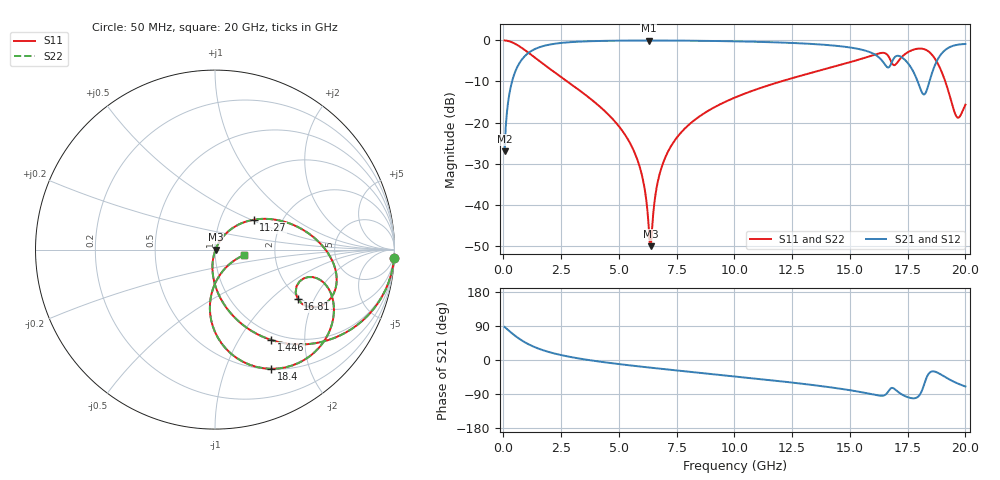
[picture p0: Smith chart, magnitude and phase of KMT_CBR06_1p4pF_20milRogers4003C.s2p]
! Data measured by Modelithics Inc. support@modelithics.com 813-866-6335
! KEMET CBR0603 1.4pF, Pad Width= 0.851mm, Pad Length= 0.64mm, Pad Gap= 0.62mm, 20mil Rogers 4003C substrate Data, January 2022
# hz S ma R 50
! 2 Port Network Data from SP1.SP block
! freq  magS11  angS11  magS21  angS21  magS12  angS12  magS22  angS22
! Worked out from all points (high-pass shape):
!   401 points, 50 MHz to 20 GHz, reference 50 ohm
!   highest |S21| = -0.03 dB at 6.284 GHz (marker M1); lowest = -27.0 dB at 50 MHz (marker M2)
!   |S21| within 3 dB of the highest: 1.087 GHz to 15.94 GHz (14.85 GHz wide, 174 % of centre); 19 GHz to end of sweep
!   lowest |S11| = -50.1 dB at 6.384 GHz (marker M3), VSWR 1.01, Z = 50.3 + j0.00703 ohm
!   |S11| at or under -10 dB: 2.763 GHz to 12.01 GHz (9.249 GHz wide, 125 % of centre); 19.13 GHz to end of sweep
!   |S22| runs from -50.1 to 0.0 dB; largest |S21 - S12| = 0
!   S11 on the Smith chart (normalised r, x): 50 MHz: 1, -42; 1.446 GHz: 0.89, -1.39; 11.27 GHz: 1.44, +0.52; 16.81 GHz: 1.94, -1.50; 18.4 GHz: 0.50, -1.45; 20 GHz: 1.38, -0.09
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5e7  0.999 -2.7  0.04465 87.3  0.04465 87.3  0.999 -2.7
4.98875e8  0.9121 -25.7  0.409 64.2  0.409 64.2  0.9121 -25.7
1.4465e9  0.5924 -58.1  0.804 31.7  0.804 31.7  0.5924 -58.1
3.391625e9  0.2348 -86.7  0.9697 2.8  0.9697 2.8  0.2348 -86.7
5.53625e9  0.0524 -101.6  0.9957 -14.6  0.9957 -14.6  0.0524 -101.6
6.035e9  0.02038 -100.1  0.9968 -18.0  0.9968 -18.0  0.02038 -100.1
6.284375e9  0.005651 -79.1  0.9969 -19.7  0.9969 -19.7  0.005651 -79.1
6.384125e9  0.003122 1.3  0.9969 -20.4  0.9969 -20.4  0.003122 1.3
6.73325e9  0.02195 59.6  0.9965 -22.6  0.9965 -22.6  0.02195 59.6
7.780625e9  0.08059 58.4  0.9933 -29.3  0.9933 -29.3  0.08059 58.4
1.0025e10  0.2018 45.6  0.9751 -43.3  0.9751 -43.3  0.2018 45.6
1.127188e10  0.272 37.7  0.9571 -51.3  0.9571 -51.3  0.272 37.7
1.336662e10  0.406 23.0  0.9054 -65.8  0.9054 -65.8  0.406 23.0
1.62095e10  0.689 -11.3  0.6372 -93.5  0.6372 -93.5  0.689 -11.3
1.670825e10  0.6136 -31.5  0.4758 -78.8  0.4758 -78.8  0.6136 -31.5
1.6808e10  0.5361 -30.8  0.5373 -73.6  0.5373 -73.6  0.5361 -30.8
1.770575e10  0.7637 -30.5  0.4381 -101.0  0.4381 -101.0  0.7637 -30.5
1.815462e10  0.7907 -51.0  0.2239 -75.1  0.2239 -75.1  0.7907 -51.0
1.8404e10  0.7339 -64.9  0.2903 -36.8  0.2903 -36.8  0.7339 -64.9
1.895262e10  0.4267 -91.7  0.6826 -38.7  0.6826 -38.7  0.4267 -91.7
1.9601e10  0.1198 -62.9  0.8796 -60.2  0.8796 -60.2  0.1198 -62.9
2e10  0.1649 -10.7  0.9045 -69.9  0.9045 -69.9  0.1649 -10.7
